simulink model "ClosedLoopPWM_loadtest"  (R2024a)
settings: Solver=FixedStepAuto  StartTime=0.0  StopTime=0.1  FixedStep=1e-7  RelTol=1e-3
undefined symbols (not defined in the file): bridge, phase, pulses, Three
libraries: spsIGBTDiodeLib x6, spsThreePhaseSeriesRLCBranchLib x6, spsDiodeLib x6, spsGroundLib x4, spsThreePhaseVIMeasurementLib x3, spsSeriesRLCBranchLib x3, spsMultimeterLib x3, spsTHDLib x2, spsabctodq0Lib x2, spsThreePhaseBreakerLib x2, slpidlib x2, spsPLL3phLib x1

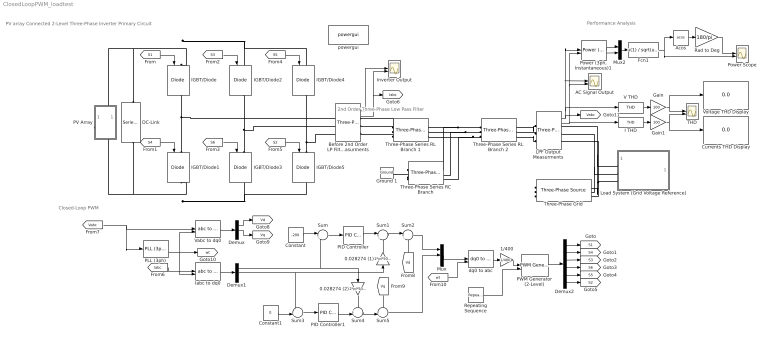
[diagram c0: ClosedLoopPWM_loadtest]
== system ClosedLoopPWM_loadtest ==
  note: Closed-Loop PWM
  note: 2nd Order Three-Phase Low Pass Filter
  note: PV array Connected 2-Level Three-Phase Inverter Primary Circuit
  note: Performance Analysis
  0.028274 (1) : Gain  Gain=2*pi*50*90e-6
  0.028274 (2) : Gain  Gain=2*pi*50*90e-6
  1/400 : Gain  Gain=1/400
  AC Signal Output : Scope  NumInputPorts=2
  Acos : Trigonometry  Operator=acos
  Before 2nd Order LP Filter Measurments : spsThreePhaseVIMeasurementLib/Three-Phase V-I Measurement  VoltageMeasurement=phase-to-phase  SetLabelV=off  LabelV=Vabc  Vpu=off  VpuLL=off  CurrentMeasurement=yes  SetLabelI=off  LabelI=Iabc  Ipu=off  Pbase=100e6  Vbase=500e3  OutputType=Complex  PhasorSimulation=off  PSBequivalent=0
  Constant : Constant  Value=-200
  Constant1 : Constant  Value=0
  Currents THD Display : Display
  DC-Link : spsSeriesRLCBranchLib/Series RLC Branch  LConnTagsString=__new0  RConnTagsString=__new0  BranchType=RC  Resistance=20e-3  Inductance=1e-3  SetiL0=off  InitialCurrent=0  Capacitance=81e-6  Setx0=off  InitialVoltage=0  Measurements=None
  Demux : Demux  Outputs=3
  Demux1 : Demux  Outputs=3
  Demux2 : Demux  Outputs=6
  Fcn1 : Fcn  Expr=u(1) / sqrt(u(1)^2 + u(2)^2)
  Gain : Gain  Gain=100
  Gain1 : Gain  Gain=100
  Ground 1 : spsGroundLib/Ground  LConnTagsString=a
  I THD : spsTHDLib/THD  Freq=50  Ts=0
  IGBT/Diode{,1..5} (6 alike) : spsIGBTDiodeLib/IGBT//Diode  Ron=1e-3  Rs=1e5  Cs=inf  Measurements=on
  Iabc to dq0 : spsabctodq0Lib/abc to dq0  Alignment=90 degrees behind phase A axis
  Inverter Output : Scope  NumInputPorts=2
  LPF Output Measurments : spsThreePhaseVIMeasurementLib/Three-Phase V-I Measurement  VoltageMeasurement=phase-to-phase  SetLabelV=off  LabelV=Vabc  Vpu=off  VpuLL=off  CurrentMeasurement=yes  SetLabelI=off  LabelI=Iabc  Ipu=off  Pbase=100e6  Vbase=500e3  OutputType=Complex  PhasorSimulation=off  PSBequivalent=0
  Load System (Grid Voltage Reference) : Subsystem
  Mux : Mux  Inputs=3
  Mux2 : Mux  Inputs=2
  PID Controller : slpidlib/PID Controller  Controller=PI  Form=Parallel  TimeDomain=Continuous-time  UseExternalTs=off  SampleTime=-1  IntegratorMethod=Forward Euler  FilterMethod=Forward Euler  ControllerParametersSource=internal  P=30  I=200  UseKiTs=off  D=0  UseExternalDerivativeSource=off  N=100  UseFilter=on  TunerSelectOption=Transfer Function Based (PID Tuner App)  InitialConditionSource=internal  InitialConditionForIntegrator=0  InitialConditionForFilter=0  DifferentiatorICPrevScaledInput=0  ExternalReset=none  TrackingMode=off  Kt=1  LimitOutput=off  SatLimitsSource=internal  UpperSaturationLimit=inf  LowerSaturationLimit=-inf  LinearizeAsGain=on  AntiWindupMode=none  Kb=1  LimitIntegrator=off  UpperIntegratorSaturationLimit=inf  LowerIntegratorSaturationLimit=-inf  POutMin=[]  POutMax=[]  IOutMin=[]  IOutMax=[]  DOutMin=[]  DOutMax=[]  NOutMin=[]  NOutMax=[]  SumOutMin=[]  SumOutMax=[]  SaturationOutMin=[]  SaturationOutMax=[]  PParamMin=[]  PParamMax=[]  IParamMin=[]  IParamMax=[]  DParamMin=[]  DParamMax=[]  NParamMin=[]  NParamMax=[]  KbParamMin=[]  KbParamMax=[]  KtParamMin=[]  KtParamMax=[]  KbOutMin=[]  KbOutMax=[]  KtOutMin=[]  KtOutMax=[]  IntegratorOutMin=[]  IntegratorOutMax=[]  FilterOutMin=[]  FilterOutMax=[]  SumI1OutMin=[]  SumI1OutMax=[]  SumI2OutMin=[]  SumI2OutMax=[]  SumI3OutMin=[]  SumI3OutMax=[]  SumI4OutMin=[]  SumI4OutMax=[]  SumDOutMin=[]  SumDOutMax=[]  DifferentiatorOutMin=[]  DifferentiatorOutMax=[]  FilterDiffOutCoefMin=[]  FilterDiffOutCoefMax=[]  ReciprocalOutMin=[]  ReciprocalOutMax=[]  SumDenOutMin=[]  SumDenOutMax=[]  SumNumOutMin=[]  SumNumOutMax=[]  DivideOutMin=[]  DivideOutMax=[]  UdiffTsProdOutMin=[]  UdiffTsProdOutMax=[]  NTsProdOutMin=[]  NTsProdOutMax=[]  UintegralTsProdOutMin=[]  UintegralTsProdOutMax=[]  UngainTsProdOutMin=[]  UngainTsProdOutMax=[]  ClampingZeroOutDataTypeStr=Inherit: Inherit via back propagation  ClampingZeroOutMin=[]  ClampingZeroOutMax=[]  FilterDenConstantOutDataTypeStr=Inherit: Inherit via back propagation  FilterDenConstantOutMin=[]  FilterDenConstantOutMax=[]  PCopyOutDataTypeStr=Inherit: Inherit via back propagation  PCopyOutMin=[]  PCopyOutMax=[]  NCopyOutDataTypeStr=Inherit: Inherit via back propagation  NCopyOutMin=[]  NCopyOutMax=[]  IntegratorContinuousStateAttributes=''  IntegratorStateMustResolveToSignalObject=off  IntegratorRTWStateStorageClass=Auto  FilterContinuousStateAttributes=''  FilterStateMustResolveToSignalObject=off  FilterRTWStateStorageClass=Auto  ParallelPVariant=InternalParameters  IdealPVariant=Disabled  IVariant=InternalParameters  DVariant=Disabled  IntegratorVariant=Continuous  SatVariant=Disabled  AWVariant=Passthrough  PCopyVariant=Disabled  TRVariant=Disabled  FdbkBlocksVariant=Forward  IdealPFdbkVariant=Disabled  SatFdbkVariant=Disabled  DerivativeFilterVariant=Disabled  NVariant=Disabled  NCopyVariant=Disabled_SignalSpec  FilterICVariant=Disabled  IntegratorICVariant=InternalICs  ExternalResetVariant=Disabled  TRSumVariant=Passthrough  SumFdbkVariant=Disabled  SumVariant=Sum_PI  TsampFilterVariant=InternalTs  TsampNgainVariant=Passthrough  TsampIntegralVariant=Disabled_SignalSpec  ExternalSaturationOutDataTypeStr=Inherit: Same as second input  DerivativeSourceVariant=Disabled
  PID Controller1 : slpidlib/PID Controller  Controller=PI  Form=Parallel  TimeDomain=Continuous-time  UseExternalTs=off  SampleTime=-1  IntegratorMethod=Forward Euler  FilterMethod=Forward Euler  ControllerParametersSource=internal  P=30  I=200  UseKiTs=off  D=0  UseExternalDerivativeSource=off  N=100  UseFilter=on  TunerSelectOption=Transfer Function Based (PID Tuner App)  InitialConditionSource=internal  InitialConditionForIntegrator=0  InitialConditionForFilter=0  DifferentiatorICPrevScaledInput=0  ExternalReset=none  TrackingMode=off  Kt=1  LimitOutput=off  SatLimitsSource=internal  UpperSaturationLimit=inf  LowerSaturationLimit=-inf  LinearizeAsGain=on  AntiWindupMode=none  Kb=1  LimitIntegrator=off  UpperIntegratorSaturationLimit=inf  LowerIntegratorSaturationLimit=-inf  POutMin=[]  POutMax=[]  IOutMin=[]  IOutMax=[]  DOutMin=[]  DOutMax=[]  NOutMin=[]  NOutMax=[]  SumOutMin=[]  SumOutMax=[]  SaturationOutMin=[]  SaturationOutMax=[]  PParamMin=[]  PParamMax=[]  IParamMin=[]  IParamMax=[]  DParamMin=[]  DParamMax=[]  NParamMin=[]  NParamMax=[]  KbParamMin=[]  KbParamMax=[]  KtParamMin=[]  KtParamMax=[]  KbOutMin=[]  KbOutMax=[]  KtOutMin=[]  KtOutMax=[]  IntegratorOutMin=[]  IntegratorOutMax=[]  FilterOutMin=[]  FilterOutMax=[]  SumI1OutMin=[]  SumI1OutMax=[]  SumI2OutMin=[]  SumI2OutMax=[]  SumI3OutMin=[]  SumI3OutMax=[]  SumI4OutMin=[]  SumI4OutMax=[]  SumDOutMin=[]  SumDOutMax=[]  DifferentiatorOutMin=[]  DifferentiatorOutMax=[]  FilterDiffOutCoefMin=[]  FilterDiffOutCoefMax=[]  ReciprocalOutMin=[]  ReciprocalOutMax=[]  SumDenOutMin=[]  SumDenOutMax=[]  SumNumOutMin=[]  SumNumOutMax=[]  DivideOutMin=[]  DivideOutMax=[]  UdiffTsProdOutMin=[]  UdiffTsProdOutMax=[]  NTsProdOutMin=[]  NTsProdOutMax=[]  UintegralTsProdOutMin=[]  UintegralTsProdOutMax=[]  UngainTsProdOutMin=[]  UngainTsProdOutMax=[]  ClampingZeroOutDataTypeStr=Inherit: Inherit via back propagation  ClampingZeroOutMin=[]  ClampingZeroOutMax=[]  FilterDenConstantOutDataTypeStr=Inherit: Inherit via back propagation  FilterDenConstantOutMin=[]  FilterDenConstantOutMax=[]  PCopyOutDataTypeStr=Inherit: Inherit via back propagation  PCopyOutMin=[]  PCopyOutMax=[]  NCopyOutDataTypeStr=Inherit: Inherit via back propagation  NCopyOutMin=[]  NCopyOutMax=[]  IntegratorContinuousStateAttributes=''  IntegratorStateMustResolveToSignalObject=off  IntegratorRTWStateStorageClass=Auto  FilterContinuousStateAttributes=''  FilterStateMustResolveToSignalObject=off  FilterRTWStateStorageClass=Auto  ParallelPVariant=InternalParameters  IdealPVariant=Disabled  IVariant=InternalParameters  DVariant=Disabled  IntegratorVariant=Continuous  SatVariant=Disabled  AWVariant=Passthrough  PCopyVariant=Disabled  TRVariant=Disabled  FdbkBlocksVariant=Forward  IdealPFdbkVariant=Disabled  SatFdbkVariant=Disabled  DerivativeFilterVariant=Disabled  NVariant=Disabled  NCopyVariant=Disabled_SignalSpec  FilterICVariant=Disabled  IntegratorICVariant=InternalICs  ExternalResetVariant=Disabled  TRSumVariant=Passthrough  SumFdbkVariant=Disabled  SumVariant=Sum_PI  TsampFilterVariant=InternalTs  TsampNgainVariant=Passthrough  TsampIntegralVariant=Disabled_SignalSpec  ExternalSaturationOutDataTypeStr=Inherit: Same as second input  DerivativeSourceVariant=Disabled
  PLL (3ph) : spsPLL3phLib/PLL (3ph)  Fmin=45  Par_Init=[0, 60]  ParK=[180, 3200, 1]  TcD=1e-4  MaxRateChangeFreq=12  FilterCutOffFreq=25  Ts=0  AGC=on
  PV Array : Subsystem
  PWM Generator (2-Level) : spsPWMGenerator2LevelLib/PWM Generator (2-Level)  ModulatorType=Three-phase bridge (6 pulses)  ModulatorMode=Synchronized  Fc=27*60  Pc=90  nF=400  MinMax="[ -1  1 ]"  SamplingTechnique=Natural  ModulatingSignals=off  m=0.8  Freq=60  Phase=0  Ts=0  ShowCarrierOutport=off
  "Power (3ph, Instantaneous)1" : spsPower3phInstantaneousLib/Power (3ph, Instantaneous)
  Power Scope : Scope  NumInputPorts=2
  Rad to Deg : Gain  Gain=180/pi
  Repeating Sequence : simulink/Sources/Repeating Sequence  rep_seq_t=[0 .00005 .0001]  rep_seq_y=[-1 1 -1]
  Sum : Sum  Inputs=|+-
  Sum1 : Sum  Inputs=|+-
  Sum2 : Sum  Inputs=|++
  Sum3 : Sum  Inputs=-+|
  Sum4 : Sum  Inputs=++|
  Sum5 : Sum  Inputs=-+|
  THD : Scope  NumInputPorts=2
  Three-Phase Series RC Branch : spsThreePhaseSeriesRLCBranchLib/Three-Phase Series RLC Branch  LConnTagsString=A|B|C  RConnTagsString=A|B|C  BranchType=RC  Resistance=20e-3  Inductance=500e-4  Capacitance=81e-6  Measurements=None
  Three-Phase Series RL Branch 1 : spsThreePhaseSeriesRLCBranchLib/Three-Phase Series RLC Branch  LConnTagsString=A|B|C  RConnTagsString=A|B|C  BranchType=RL  Resistance=20e-3  Inductance=45e-6  Capacitance=1e-6  Measurements=None
  Three-Phase Series RL Branch 2 : spsThreePhaseSeriesRLCBranchLib/Three-Phase Series RLC Branch  LConnTagsString=A|B|C  RConnTagsString=A|B|C  BranchType=RL  Resistance=20e-3  Inductance=45e-6  Capacitance=1e-6  Measurements=None
  Three-Phase Grid : spsThreePhaseSourceLib/Three-Phase Source  InternalConnection=Yg  VoltagePhases=off  Voltage=240  PhaseAngle=0  Voltage_phases=[25e3 25e3 25e3]/sqrt(3)  PhaseAngles_phases=[0 -120 +120]  Frequency=50  NonIdealSource=on  SpecifyImpedance=off  Resistance=.001e-3  Inductance=.001e-9  ShortCircuitLevel=100e6  BaseVoltage=240  XRratio=7  BusType=swing  Pref=10e3  Qref=0  Prefabc=[10e3, 10e3, 10e3]  Qrefabc=[0, 0, 0]  Qmin=-inf  Qmax=inf
  V THD : spsTHDLib/THD  Freq=50  Ts=0
  Vabc to dq0 : spsabctodq0Lib/abc to dq0  Alignment=90 degrees behind phase A axis
  Voltage THD Display : Display
  dq0 to abc : spsdq0toabcLib/dq0 to abc  Alignment=90 degrees behind phase A axis
  powergui : spspowerguiLib/powergui  Priority=1  SimulationMode=Discrete  SampleTime=1e-6  frequency=60  Iterations=50  frequencyindice=0  Pbase=100e6  ErrMax=1e-4  UnitsV=kV  UnitsW=MW  buscounter=0  FunctionMessages=off  echomessages=off  EnableUseOfTLC=off  CurrentSourceSwitches=off  DisableSnubberDevices=off  DisableRonSwitches=off  DisableVfSwitches=off  DisplayEquations=off  AutomaticDiscreteSolvers=off  SolverType=Tustin/Backward Euler (TBE)  Interpol=off  ExternalGateDelay=off  methode=off  Ts=100  x0status=blocks  SPID=on  SwTol=0  HookPort=off  NonlinearTolerance=1e-4  nMaxIteration=100  ContinueOnMaxIteration=off  RestoreLinks=warning  ResistiveCurrentMeasurement=off  Frange=[0:2:500]  Ylog=off  Xlog=on  ShowGrid=off  save=off  variable=ZData  structure=0  ZoomFFT=off  StartTime=0.0  cycles=1  DisplayStyle=1  fundamental=60  FreqAxis=off  MaxFrequency=1000  frequencyindicesteady=1  RmsSteady=1  display=off
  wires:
  [S1] -> IGBT/Diode/1
  [S6] -> IGBT/Diode3/1
  [S5] -> IGBT/Diode4/1
  [S2] -> IGBT/Diode5/1
  [S3] -> IGBT/Diode2/1
  [S4] -> IGBT/Diode1/1
  Before 2nd Order LP Filter Measurments/2 -> Inverter Output/2, [Iabc]
  Before 2nd Order LP Filter Measurments/1 -> Inverter Output/1
  [Iabc] -> Iabc to dq0/1
  [Vabc] -> Vabc to dq0/1, PLL (3ph)/1
  PLL (3ph)/2 -> Iabc to dq0/2, Vabc to dq0/2, [wt]
  Vabc to dq0/1 -> Demux/1
  Demux/1 -> [Vd]
  Demux/2 -> [Vq]
  Iabc to dq0/1 -> Demux1/1
  Sum/1 -> PID Controller/1
  Sum1/1 -> Sum2/1
  PID Controller/1 -> Sum1/1
  Constant/1 -> Sum/1
  Demux1/1 -> 0.028274 (2)/1, Sum/2
  Sum3/1 -> PID Controller1/1
  Constant1/1 -> Sum3/2
  Demux1/2 -> 0.028274 (1)/1, Sum3/1
  PID Controller1/1 -> Sum4/2
  Sum4/1 -> Sum5/2
  0.028274 (1)/1 -> Sum1/2
  0.028274 (2)/1 -> Sum4/1
  [Vd] -> Sum2/2
  [Vq] -> Sum5/1
  Mux/1 -> dq0 to abc/1
  Sum5/1 -> Mux/2
  Sum2/1 -> Mux/1
  [wt] -> dq0 to abc/2
  dq0 to abc/1 -> 1/400/1
  Repeating Sequence/1 -> PWM Generator (2-Level)/2
  PWM Generator (2-Level)/1 -> Demux2/1
  Demux2/6 -> [S2]
  Demux2/5 -> [S5]
  Demux2/4 -> [S6]
  Demux2/3 -> [S3]
  Demux2/2 -> [S4]
  Demux2/1 -> [S1]
  1/400/1 -> PWM Generator (2-Level)/1
  V THD/1 -> Gain/1
  I THD/1 -> Gain1/1
  Gain/1 -> Voltage THD Display/1, THD/1
  Gain1/1 -> THD/2, Currents THD Display/1
  Rad to Deg/1 -> Power Scope/1
  LPF Output Measurments/1 -> "Power (3ph, Instantaneous)1"/1, AC Signal Output/1, V THD/1, [Vabc]
  Fcn1/1 -> Power Scope/2, Acos/1
  Acos/1 -> Rad to Deg/1
  LPF Output Measurments/2 -> I THD/1, "Power (3ph, Instantaneous)1"/2, AC Signal Output/2
  "Power (3ph, Instantaneous)1"/1 -> Mux2/1
  Mux2/1 -> Fcn1/1
  "Power (3ph, Instantaneous)1"/2 -> Mux2/2
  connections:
  IGBT/Diode5/LConn1 -- IGBT/Diode4/RConn1 -- Before 2nd Order LP Filter Measurments/LConn3
  DC-Link/LConn1 -- PV Array/LConn1 -- IGBT/Diode/LConn1 -- IGBT/Diode4/LConn1 -- IGBT/Diode2/LConn1
  IGBT/Diode3/LConn1 -- Before 2nd Order LP Filter Measurments/LConn2 -- IGBT/Diode2/RConn1
  IGBT/Diode1/LConn1 -- IGBT/Diode/RConn1 -- Before 2nd Order LP Filter Measurments/LConn1
  Three-Phase Series RL Branch 1/LConn1 -- Before 2nd Order LP Filter Measurments/RConn1
  Three-Phase Series RL Branch 1/LConn3 -- Before 2nd Order LP Filter Measurments/RConn3
  Three-Phase Series RL Branch 1/LConn2 -- Before 2nd Order LP Filter Measurments/RConn2
  Three-Phase Series RL Branch 2/LConn1 -- Three-Phase Series RC Branch/LConn1 -- Three-Phase Series RL Branch 1/RConn1
  Three-Phase Series RL Branch 2/LConn2 -- Three-Phase Series RC Branch/LConn2 -- Three-Phase Series RL Branch 1/RConn2
  Three-Phase Series RL Branch 2/LConn3 -- Three-Phase Series RC Branch/LConn3 -- Three-Phase Series RL Branch 1/RConn3
  Three-Phase Series RC Branch/RConn1 -- Three-Phase Series RC Branch/RConn3 -- Three-Phase Series RC Branch/RConn2 -- Ground 1/LConn1
  LPF Output Measurments/LConn2 -- Three-Phase Series RL Branch 2/RConn2
  LPF Output Measurments/LConn1 -- Three-Phase Series RL Branch 2/RConn1
  LPF Output Measurments/LConn3 -- Three-Phase Series RL Branch 2/RConn3
  DC-Link/RConn1 -- PV Array/RConn1 -- IGBT/Diode5/RConn1 -- IGBT/Diode3/RConn1 -- IGBT/Diode1/RConn1
  LPF Output Measurments/RConn1 -- Three-Phase Grid/RConn1 -- Load System (Grid Voltage Reference)/LConn1
  LPF Output Measurments/RConn2 -- Three-Phase Grid/RConn2 -- Load System (Grid Voltage Reference)/LConn2
  Three-Phase Grid/RConn3 -- Load System (Grid Voltage Reference)/LConn3 -- LPF Output Measurments/RConn3

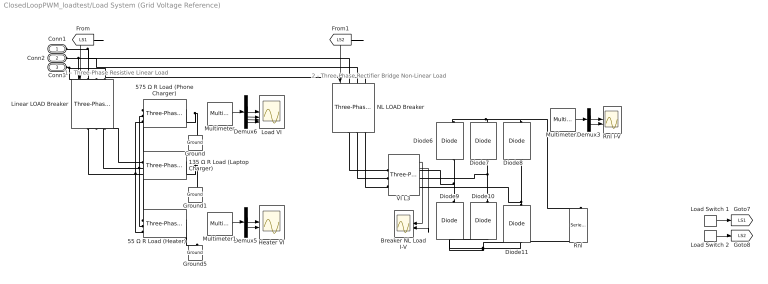
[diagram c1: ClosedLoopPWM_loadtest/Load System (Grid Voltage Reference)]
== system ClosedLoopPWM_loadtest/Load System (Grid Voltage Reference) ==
  note: 1 - Three-Phase Resistive Linear Load
  note: 2 - Three-Phase Rectifier Bridge Non-Linear Load
  135 Ω R Load (Laptop Charger) : spsThreePhaseSeriesRLCBranchLib/Three-Phase Series RLC Branch  LConnTagsString=A|B|C  RConnTagsString=A|B|C  BranchType=R  Resistance=135  Inductance=5.1e-3  Capacitance=1e-6  Measurements=Branch voltages and currents
  55 Ω R Load (Heater) : spsThreePhaseSeriesRLCBranchLib/Three-Phase Series RLC Branch  LConnTagsString=A|B|C  RConnTagsString=A|B|C  BranchType=R  Resistance=55  Inductance=5.1e-3  Capacitance=1e-6  Measurements=Branch voltages and currents
  575 Ω R Load (Phone Charger) : spsThreePhaseSeriesRLCBranchLib/Three-Phase Series RLC Branch  LConnTagsString=A|B|C  RConnTagsString=A|B|C  BranchType=R  Resistance=575  Inductance=5.1e-3  Capacitance=1e-6  Measurements=Branch voltages and currents
  Breaker NL Load I-V : Scope  NumInputPorts=2
  Demux3 : Demux  Outputs=2
  Demux5 : Demux  Outputs=2
  Demux6 : Demux
  Diode{6..11} (6 alike) : spsDiodeLib/Diode  Ron=0.001  Lon=0  Vf=0.8  IC=0  UseSnubber=0  Rs=10e+6  Cs=250e-9  Measurements=off
  Ground : spsGroundLib/Ground  LConnTagsString=a
  Ground1 : spsGroundLib/Ground  LConnTagsString=a
  Ground5 : spsGroundLib/Ground  LConnTagsString=a
  Heater VI : Scope  NumInputPorts=2
  Linear LOAD Breaker : spsThreePhaseBreakerLib/Three-Phase Breaker  InitialState=open  SwitchA=on  SwitchB=on  SwitchC=on  SwitchTimes="[1/60  5/60]"  External=on  BreakerResistance=0.01  SnubberResistance=1e6  SnubberCapacitance=inf  Measurements=None
  Load Switch 1 : DiscretePulseGenerator  PulseType=Time based  Period=0.1  PulseWidth=50
  Load Switch 2 : DiscretePulseGenerator  PulseType=Time based  Period=0.1  PulseWidth=50  PhaseDelay=0.05
  Load VI : Scope  NumInputPorts=4
  Multimeter : spsMultimeterLib/Multimeter  L=20  sel=[8 2 18 12]  yselected={}  Gain=[1 1 1 1]  OutputType=Complex  PlotAtSimulationStop=off  PhasorSimulation=off
  Multimeter1 : spsMultimeterLib/Multimeter  L=20  sel=[5 15]  yselected={}  Gain=[1 1]  OutputType=Complex  PlotAtSimulationStop=off  PhasorSimulation=off
  Multimeter2 : spsMultimeterLib/Multimeter  L=20  sel=[1 11]  yselected={}  Gain=[1 1]  OutputType=Complex  PlotAtSimulationStop=off  PhasorSimulation=off
  NL LOAD Breaker : spsThreePhaseBreakerLib/Three-Phase Breaker  InitialState=open  SwitchA=on  SwitchB=on  SwitchC=on  SwitchTimes="[1/60  5/60]"  External=on  BreakerResistance=0.01  SnubberResistance=1e6  SnubberCapacitance=inf  Measurements=None
  Rnl : spsSeriesRLCBranchLib/Series RLC Branch  LConnTagsString=__new0  RConnTagsString=__new0  BranchType=R  Resistance=60  Inductance=1e-6  SetiL0=off  InitialCurrent=0  Capacitance=0.01598  Setx0=off  InitialVoltage=0  Measurements=Branch voltage and current
  Rnl I-V : Scope  NumInputPorts=2
  VI L3 : spsThreePhaseVIMeasurementLib/Three-Phase V-I Measurement  VoltageMeasurement=phase-to-phase  SetLabelV=off  LabelV=Vabc  Vpu=off  VpuLL=off  CurrentMeasurement=yes  SetLabelI=off  LabelI=Iabc  Ipu=off  Pbase=100e6  Vbase=500e3  OutputType=Complex  PhasorSimulation=off  PSBequivalent=0
  Conn1 : PMIOPort  Side=Left
  Conn2 : PMIOPort  Port=2  Side=Left
  Conn3 : PMIOPort  Port=3  Side=Left
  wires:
  Demux5/2 -> Heater VI/2
  Demux6/2 -> Load VI/2
  Demux6/4 -> Load VI/4
  Demux6/1 -> Load VI/1
  Multimeter/1 -> Demux6/1
  Demux6/3 -> Load VI/3
  Demux5/1 -> Heater VI/1
  Multimeter1/1 -> Demux5/1
  Load Switch 1/1 -> [LS1]
  Load Switch 2/1 -> [LS2]
  [LS1] -> Linear LOAD Breaker/1
  [LS2] -> NL LOAD Breaker/1
  Multimeter2/1 -> Demux3/1
  Demux3/1 -> Rnl I-V/1
  Demux3/2 -> Rnl I-V/2
  VI L3/2 -> Breaker NL Load I-V/2
  VI L3/1 -> Breaker NL Load I-V/1
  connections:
  55 Ω R Load (Heater)/LConn2 -- 135 Ω R Load (Laptop Charger)/LConn2 -- Linear LOAD Breaker/RConn2 -- 575 Ω R Load (Phone Charger)/LConn2
  55 Ω R Load (Heater)/LConn3 -- 135 Ω R Load (Laptop Charger)/LConn3 -- Linear LOAD Breaker/RConn3 -- 575 Ω R Load (Phone Charger)/LConn3
  55 Ω R Load (Heater)/RConn1 -- 55 Ω R Load (Heater)/RConn2 -- 55 Ω R Load (Heater)/RConn3 -- Ground5/LConn1
  55 Ω R Load (Heater)/LConn1 -- 135 Ω R Load (Laptop Charger)/LConn1 -- Linear LOAD Breaker/RConn1 -- 575 Ω R Load (Phone Charger)/LConn1
  575 Ω R Load (Phone Charger)/RConn1 -- Ground/LConn1 -- 575 Ω R Load (Phone Charger)/RConn3 -- 575 Ω R Load (Phone Charger)/RConn2
  135 Ω R Load (Laptop Charger)/RConn1 -- Ground1/LConn1 -- 135 Ω R Load (Laptop Charger)/RConn3 -- 135 Ω R Load (Laptop Charger)/RConn2
  Conn1/RConn1 -- NL LOAD Breaker/LConn1 -- Linear LOAD Breaker/LConn1
  Conn2/RConn1 -- NL LOAD Breaker/LConn2 -- Linear LOAD Breaker/LConn2
  Conn3/RConn1 -- NL LOAD Breaker/LConn3 -- Linear LOAD Breaker/LConn3
  Rnl/LConn1 -- Diode8/RConn1 -- Diode6/RConn1 -- Diode7/RConn1
  Diode9/RConn1 -- VI L3/RConn1 -- Diode6/LConn1
  Diode11/RConn1 -- VI L3/RConn3 -- Diode8/LConn1
  Diode9/LConn1 -- Rnl/RConn1 -- Diode11/LConn1 -- Diode10/LConn1
  Diode7/LConn1 -- Diode10/RConn1 -- VI L3/RConn2
  NL LOAD Breaker/RConn1 -- VI L3/LConn1
  NL LOAD Breaker/RConn2 -- VI L3/LConn2
  NL LOAD Breaker/RConn3 -- VI L3/LConn3

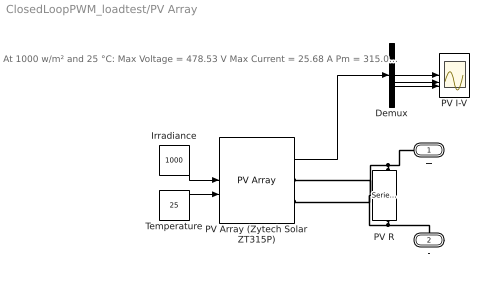
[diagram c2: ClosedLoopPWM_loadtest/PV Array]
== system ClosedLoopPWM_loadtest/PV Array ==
  note: At 1000 w/m² and 25 °C: Max Voltage = 478.53 V Max Current = 25.68 A Pm = 315.0936
  Demux : Demux  Outputs=5
  Irradiance : Constant  Value=1000
  PV I-V : Scope  NumInputPorts=5
  PV Array (Zytech Solar ZT315P) : spsPVArrayLib/PV Array  Npar=3  Nser=13  PlotType=array @ 25 deg.C & specified irradiances  S_vec="[ 1000  500  100 ]"  Temp_C_vec="[ 45 25  ]"  ModuleName=Zytech Solar ZT315P  PlotWhenSelected=off  Pm=315.0936  Ncell=72  Voc=46.44  Isc=9.01  Vm=36.81  Im=8.56  beta_Voc_pc=-0.3199  alpha_Isc_pc=0.048302  beta_Voc=-0.14856  alpha_Isc=0.004352  IL=9.0792  I0=6.901e-11  nI=0.9809  Rsh=572.7811  Rs=0.50125  RobustModel=off  RobustCellTemperature=313.3991  BAL=on  Tc=1e-6  Tfilter=5e-5
  PV R : spsSeriesRLCBranchLib/Series RLC Branch  LConnTagsString=__new0  RConnTagsString=__new0  BranchType=R  Resistance=17.2  Inductance=1e-3  SetiL0=off  InitialCurrent=0  Capacitance=1e-6  Setx0=off  InitialVoltage=0  Measurements=None
  Temperature : Constant  Value=25
  + : PMIOPort  Side=Left
  - : PMIOPort  Port=2  Side=Right
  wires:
  Irradiance/1 -> PV Array (Zytech Solar ZT315P)/1
  Temperature/1 -> PV Array (Zytech Solar ZT315P)/2
  PV Array (Zytech Solar ZT315P)/1 -> Demux/1
  Demux/3 -> PV I-V/3
  Demux/2 -> PV I-V/2
  Demux/1 -> PV I-V/1
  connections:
  PV R/LConn1 -- +/RConn1 -- PV Array (Zytech Solar ZT315P)/RConn1
  PV R/RConn1 -- -/RConn1 -- PV Array (Zytech Solar ZT315P)/RConn2
